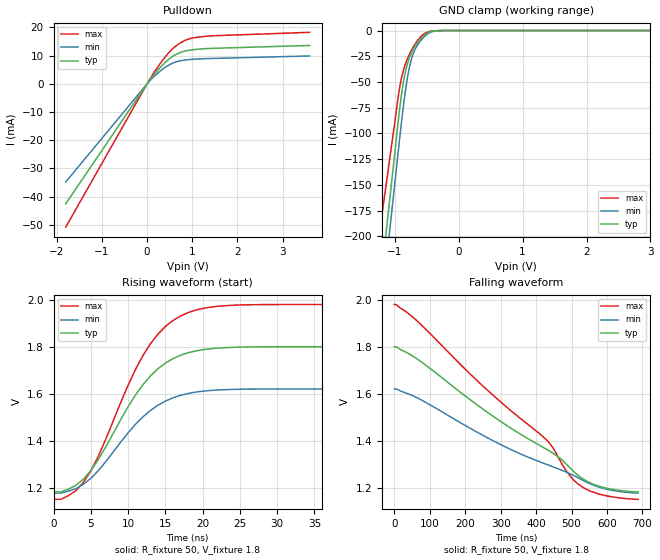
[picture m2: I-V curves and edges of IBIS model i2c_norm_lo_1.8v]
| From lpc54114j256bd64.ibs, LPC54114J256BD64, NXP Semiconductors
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[Model]   i2c_norm_lo_1.8v
Model_type I/O_open_drain
Vinl=4.000E-01
Vinh=1.500E+00
Vref=1.800E+00
Rref=1.000E+03
Cref=0.000E+00
Vmeas=9.000E-01
C_comp   1.270E-12   1.260E-12   1.280E-12
[Voltage Range]   1.800E+00   1.620E+00   1.980E+00
[POWER Clamp Reference]   1.800E+00   1.620E+00   1.980E+00
[GND Clamp Reference]   0.000E+00   0.000E+00   0.000E+00
[Pullup Reference]   1.800E+00   1.620E+00   1.980E+00
[Pulldown Reference]   0.000E+00   0.000E+00   0.000E+00
[Temperature Range]   25   105   -40
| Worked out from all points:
|   slope of the pulldown table from 0 to 0.27 V, typ, clamps not added: 49.6 ohm
|   GND clamp passes 1 mA (typ) near -0.43 V on its own axis
|   rising waveform, R_fixture 50, V_fixture 1.8: 20-80 % time 7.31ns typ, 7.33ns min, 7.31ns max; typ from 1.18 V to 1.8 V
|   falling waveform, R_fixture 50, V_fixture 1.8: 20-80 % time 354ns typ, 361ns min, 339ns max; typ from 1.8 V to 1.18 V
[GND Clamp]
-1.8V     -573.5mA   -607.6mA   -447mA
-1.02V    -130mA     -159.7mA   -97.63mA
-940mV    -84.16mA   -113.8mA   -61.27mA
-880mV    -55.56mA   -80.46mA   -41.97mA
-840mV    -41.64mA   -60.98mA   -33.55mA
-780mV    -27.9mA    -38.28mA   -24.3mA
-740mV    -21.73mA   -27.91mA   -19.22mA
-680mV    -14.85mA   -17.95mA   -12.82mA
-520mV    -3.516mA   -4.832mA   -2.394mA
-400mV    -588.2uA   -942.1uA   -363.9uA
-240mV    0A         0A         0A
3.6V      0A         0A         0A
[Pulldown]
-1.8V     -42.51mA   -34.77mA   -50.8mA
80mV      1.77mA     1.408mA    2.159mA
380mV     7.306mA    5.641mA    9.148mA
600mV     10.1mA     7.572mA    12.95mA
840mV     11.68mA    8.469mA    15.46mA
980mV     12.05mA    8.698mA    16.23mA
1.16V     12.36mA    8.87mA     16.64mA
1.4V      12.58mA    9.005mA    17.03mA
3.6V      13.63mA    9.91mA     18.29mA
[Rising Waveform]
R_fixture = 50
V_fixture = 1.8
V_fixture_min = 1.62
V_fixture_max = 1.98
0s        1.181V     1.176V     1.15V
2ns       1.193V     1.185V     1.166V
4ns       1.236V     1.213V     1.222V
6ns       1.319V     1.272V     1.333V
10ns      1.544V     1.433V     1.636V
12ns      1.639V     1.501V     1.763V
14ns      1.706V     1.551V     1.854V
17ns      1.763V     1.593V     1.931V
24ns      1.797V     1.618V     1.977V
56ns      1.8V       1.62V      1.98V
[Falling Waveform]
R_fixture = 50
V_fixture = 1.8
V_fixture_min = 1.62
V_fixture_max = 1.98
0s        1.8V       1.62V      1.98V
54ns      1.758V     1.59V      1.924V
247ns     1.538V     1.425V     1.637V
429ns     1.363V     1.299V     1.403V
448ns     1.346V     1.288V     1.368V
486ns     1.299V     1.265V     1.269V
518ns     1.252V     1.242V     1.216V
547ns     1.224V     1.219V     1.189V
585ns     1.202V     1.199V     1.169V
688ns     1.181V     1.176V     1.15V
[Ramp]
dV/dt_r   3.7126E-01/7.2920E-09   2.6611E-01/7.3020E-09   4.9817E-01/7.2900E-09
dV/dt_f   3.7126E-01/3.5425E-07   2.6611E-01/3.6087E-07   4.9817E-01/3.3887E-07
R_load = 50
